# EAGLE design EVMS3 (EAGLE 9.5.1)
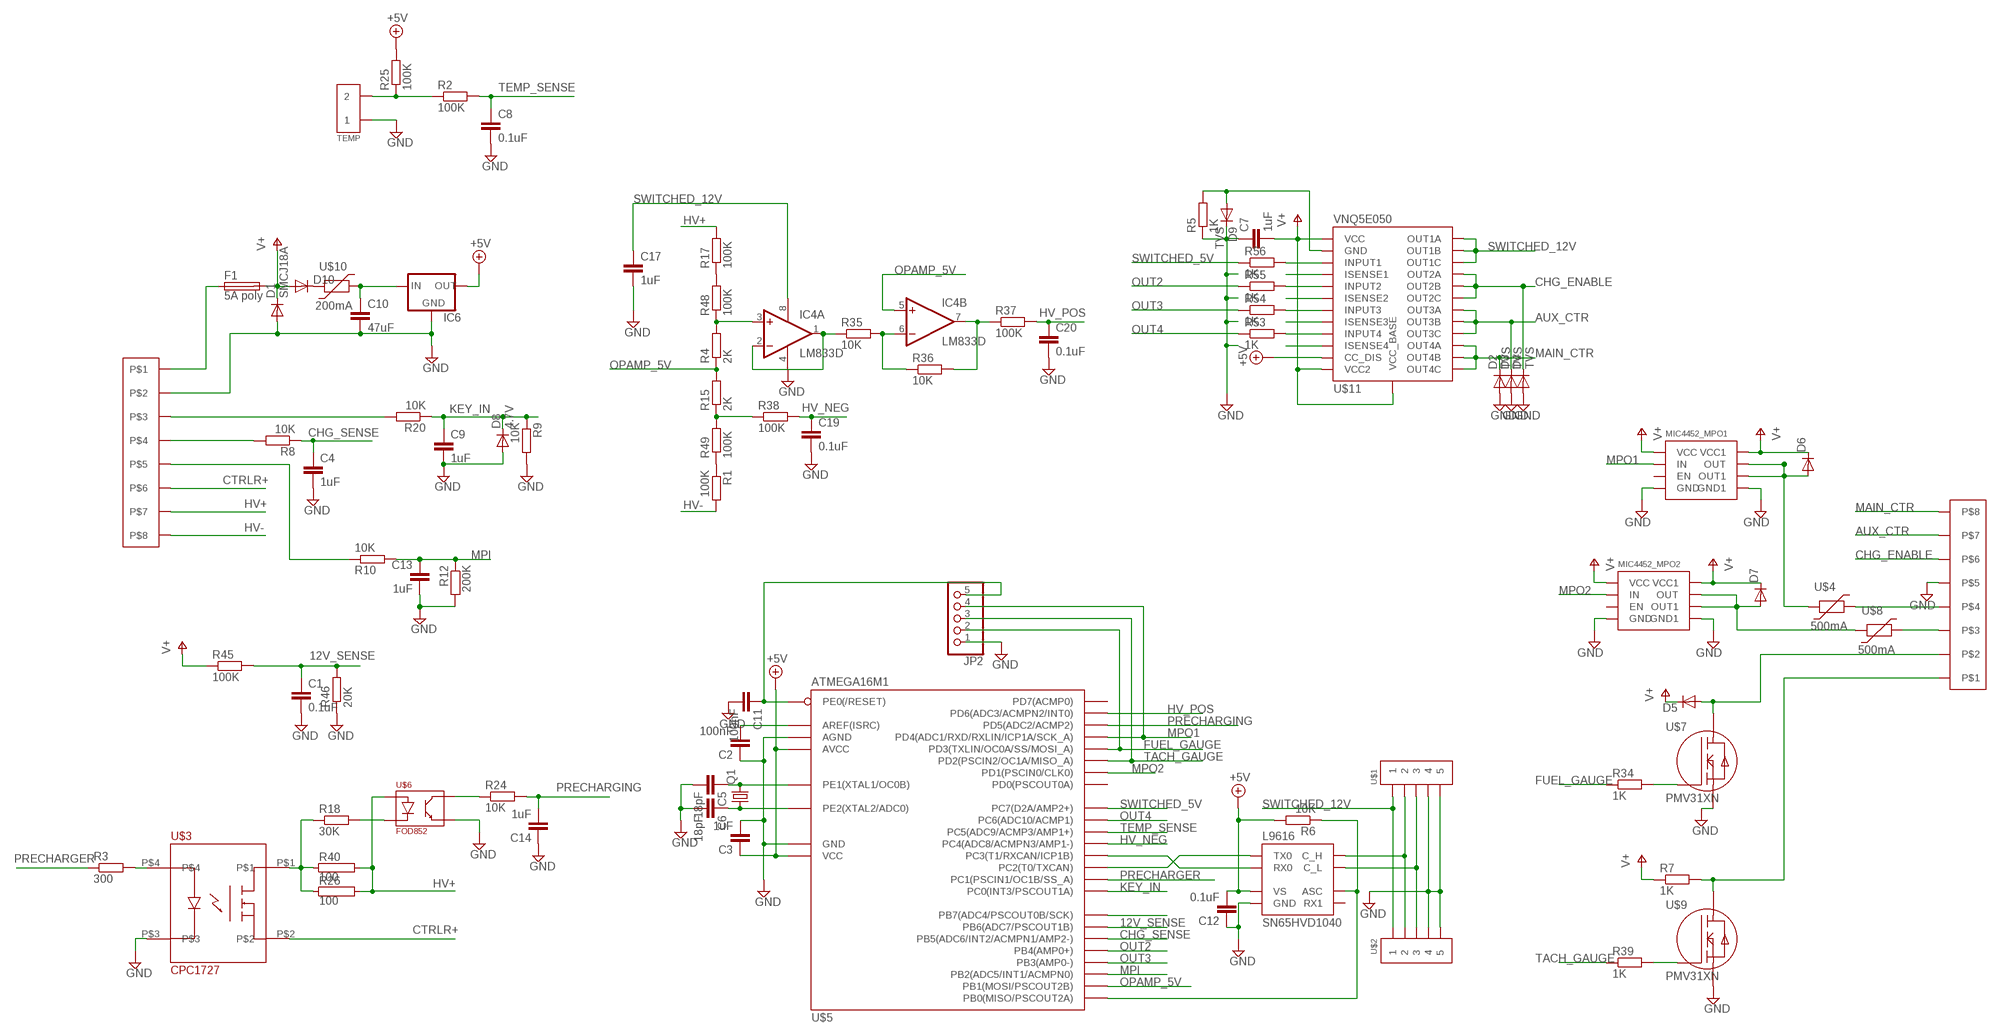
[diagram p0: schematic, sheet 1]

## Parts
C1  0.1uF  C-EUC1206  [C1206]
C2  100nF  C-EUC1206  [C1206]
C3  1uF  C-EUC1206  [C1206]
C4  1uF  C-EUC1206  [C1206]
C5  18pF  C-EUC0805  [C0805]
C6  18pF  C-EUC0805  [C0805]
C7  1uF  C-EUC1206  [C1206]
C8  0.1uF  C-EUC1206  [C1206]
C9  1uF  C-EUC1206  [C1206]
C10  47uF  C-EUC1206  [C1206]
C11  100nF  C-EUC1206  [C1206]
C12  0.1uF  C-EUC1206  [C1206]
C13  1uF  C-EUC1206  [C1206]
C14  1uF  C-EUC1206  [C1206]
C17  1uF  C-EUC1206  [C1206]
C19  0.1uF  C-EUC1206  [C1206]
C20  0.1uF  C-EUC1206  [C1206]
D1  SMCJ18A  DIODE-SMC  [SMC]
D2  TVS  DIODE-SOD123  [SOD123]
D3  TVS  DIODE-SOD123  [SOD123]
D4  TVS  DIODE-SOD123  [SOD123]
D5  DIODE-SOD123  [SOD123]
D6  DIODE-SOD123  [SOD123]
D7  DIODE-SOD123  [SOD123]
D8  4.7V  DIODE-SOD123  [SOD123]
D9  TVS  DIODE-SOD123  [SOD123]
D10  DIODE-SOD123  [SOD123]
F1  5A poly  TE5  [TE5]
IC4  LM833D  [SO08]
IC6  78LXXSOT89  [SOT89R]
JP2  PINHD-1X5  [1X05]
MIC4452_MPO1  IXDD414CI  [SOIC8]
MIC4452_MPO2  IXDD414CI  [SOIC8]
Q1  CRYSTALCTS406  [CTS406]
R1  100K  R-EU_R1206  [R1206]
R2  100K  R-EU_R1206  [R1206]
R3  300  R-EU_R1206  [R1206]
R4  2K  R-EU_R1206  [R1206]
R5  1K  R-EU_R1206  [R1206]
R6  10K  R-EU_R1206  [R1206]
R7  1K  R-EU_R1206  [R1206]
R8  10K  R-EU_R1206  [R1206]
R9  10K  R-EU_R1206  [R1206]
R10  10K  R-EU_R1206  [R1206]
R12  200K  R-EU_R1206  [R1206]
R15  2K  R-EU_R1206  [R1206]
R17  100K  R-EU_R1206  [R1206]
R18  30K  R-EU_R2512  [R2512]
R20  10K  R-EU_R1206  [R1206]
R24  10K  R-EU_R1206  [R1206]
R25  100K  R-EU_R1206  [R1206]
R26  100  RKH206-8  [KH206-8]
R34  1K  R-EU_R1206  [R1206]
R35  10K  R-EU_R1206  [R1206]
R36  10K  R-EU_R1206  [R1206]
R37  100K  R-EU_R1206  [R1206]
R38  100K  R-EU_R1206  [R1206]
R39  1K  R-EU_R1206  [R1206]
R40  100  RKH206-8  [KH206-8]
R45  100K  R-EU_R1206  [R1206]
R46  20K  R-EU_R1206  [R1206]
R48  100K  R-EU_R1206  [R1206]
R49  100K  R-EU_R1206  [R1206]
R53  1K  R-EU_R1206  [R1206]
R54  1K  R-EU_R1206  [R1206]
R55  1K  R-EU_R1206  [R1206]
R56  1K  R-EU_R1206  [R1206]
SN65HVD1040  L9616  [SOIC8]
TEMP  MOLEX-39502-1002  [MOLEX-39502-1002]
U$1  MOLEX-39502-1005  [MOLEX-39502-1005]
U$2  MOLEX-39502-1005  [MOLEX-39502-1005]
U$3  CPC1727  [CPC1727]
U$4  500mA  1206_POLYSWITCH  [1206]
U$5  ATMEGA16M1  [TQFP32]
U$6  FOD852  [SMD4]
U$7  PMV31XN  [SOT23]
U$8  500mA  1206_POLYSWITCH  [1206]
U$9  PMV31XN  [SOT23]
U$10  200mA  1206_POLYSWITCH  [1206]
U$11  VNQ5E050  [POWERSSO-24]
U$12  MOLEX-38720-6208INLINE_PINS  [MOLEX-38720-6208-B]
U$13  MOLEX-38720-6208INLINE_PINS  [MOLEX-38720-6208-B]

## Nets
12V_SENSE: C1.1 R45.2 R46.2 U$5.27(PB6(ADC7/PSCOUT1B))
+5V: C3.1 C12.2 IC6.2(OUT) R6.2 R25.2 SN65HVD1040.P$3(VS) U$5.4(VCC) U$5.19(AVCC) U$11.P$11(CC_DIS)
AUX_CTR: D3.C U$11.P$16(OUT3C) U$11.P$17(OUT3B) U$11.P$18(OUT3A) U$13.7
CHG_ENABLE: D4.C U$11.P$19(OUT2C) U$11.P$20(OUT2B) U$11.P$21(OUT2A) U$13.6
CHG_SENSE: C4.1 R8.1 U$5.26(PB5(ADC6/INT2/ACMPN1/AMP2-))
CTRLR+: U$3.P$2 U$12.6
FSA: R6.1 SN65HVD1040.P$8(ASC) U$5.8(PB0(MISO/PSCOUT2A))
FUEL_GAUGE: JP2.2 R34.1 U$5.2(PD3(TXLIN/OC0A/SS/MOSI_A))
GND: C1.2 C2.1 C3.2 C4.2 C5.2 C6.2 C7.1 C8.2 C9.2 C10.2 C11.2 C12.1 C13.2 C14.1 C17.2 C19.2 C20.2 D1.A D2.A D3.A D4.A D8.A D9.C IC4.4(P:V-) IC6.4(GND) JP2.1 MIC4452_MPO1.P$4(GND) MIC4452_MPO1.P$5(GND1) MIC4452_MPO2.P$4(GND) MIC4452_MPO2.P$5(GND1) R5.1 R9.2 R12.2 R46.1 SN65HVD1040.P$2(GND) TEMP.1 U$1.4 U$1.5 U$2.4 U$2.5 U$3.P$3 U$5.5(GND) U$5.20(AGND) U$6.P$3(EM) U$7.P$2(S) U$9.P$2(S) U$12.2 U$13.5
HV+: R17.2 R26.2 R40.2 U$6.P$1(AN) U$12.7
HV-: R1.2 U$12.8
HV_NEG: C19.1 R38.2 U$5.17(PC4(ADC8/ACMPN3/AMP1-))
HV_POS: C20.1 R37.2 U$5.14(PD6(ADC3/ACMPN2/INT0))
KEY_IN: C9.1 D8.C R9.1 R20.1 U$5.30(PC0(INT3/PSCOUT1A))
MAIN_CTR: D2.C U$11.P$13(OUT4C) U$11.P$14(OUT4B) U$11.P$15(OUT4A) U$13.8
MPI: C13.1 R10.2 R12.1 U$5.16(PB2(ADC5/INT1/ACMPN0))
MPO1: JP2.4 MIC4452_MPO1.P$2(IN) U$5.12(PD4(ADC1/RXD/RXLIN/ICP1A/SCK_A))
MPO2: MIC4452_MPO2.P$2(IN) U$5.32(PD1(PSCIN0/CLK0))
N$1: IC4.3(A:+IN) R4.2 R48.1
N$2: D9.A R5.2 U$11.P$2(GND)
N$3: C10.1 IC6.1(IN) U$10.P$2
N$4: U$4.P$2 U$13.4
N$5: R2.1 R25.1 TEMP.2
N$6: U$5.28(PB7(ADC4/PSCOUT0B/SCK))
N$7: SN65HVD1040.P$6(C_L) U$1.3 U$2.3
N$8: U$11.P$4(ISENSE1)
N$9: R18.2 U$6.P$2(CAT)
N$10: SN65HVD1040.P$7(C_H) U$1.2 U$2.2
N$11: F1.1 U$12.1
N$12: SN65HVD1040.P$1(TX0) U$5.6(PC2(T0/TXCAN))
N$13: R10.1 U$12.5
N$14: R15.1 R38.1 R49.2
N$15: D10.C U$10.P$1
N$16: R24.1 U$6.P$4(COL)
N$17: SN65HVD1040.P$4(RX0) U$5.7(PC3(T1/RXCAN/ICP1B))
N$18: U$11.P$6(ISENSE2)
N$19: U$8.P$2 U$13.3
N$21: C6.1 Q1.1 U$5.11(PE2(XTAL2/ADC0))
N$22: D6.A MIC4452_MPO1.P$6(OUT) MIC4452_MPO1.P$7(OUT1) U$4.P$1
N$25: U$11.P$8(ISENSE3)
N$26: R18.1 R26.1 R40.1 U$3.P$1
N$27: R1.1 R49.1
N$28: U$11.P$10(ISENSE4)
N$30: R3.2 U$3.P$4
N$31: R17.1 R48.2
N$32: R20.2 U$12.3
N$34: C5.1 Q1.3 U$5.10(PE1(XTAL1/OC0B))
N$35: R53.2 U$11.P$9(INPUT4)
N$37: R8.2 U$12.4
N$39: R54.2 U$11.P$7(INPUT3)
N$41: R55.2 U$11.P$5(INPUT2)
N$42: C2.2 U$5.21(AREF(ISRC))
N$43: R56.2 U$11.P$3(INPUT1)
N$44: C11.1 JP2.5 U$5.31(PE0(/RESET))
N$51: D7.A MIC4452_MPO2.P$6(OUT) MIC4452_MPO2.P$7(OUT1) U$8.P$1
N$54: D5.A U$7.P$3(D) U$13.2
N$55: R34.2 U$7.P$1(G)
N$56: R7.2 U$9.P$3(D) U$13.1
N$57: R39.2 U$9.P$1(G)
N$64: IC4.1(A:OUT) IC4.2(A:-IN) R35.1
N$65: IC4.6(B:-IN) R35.2 R36.1
N$66: IC4.7(B:OUT) R36.2 R37.1
OPAMP_5V: IC4.5(B:+IN) R4.1 R15.2 U$5.9(PB1(MOSI/PSCOUT2B))
OUT2: R55.1 U$5.24(PB4(AMP0+))
OUT3: R54.1 U$5.23(PB3(AMP0-))
OUT4: R53.1 U$5.22(PC6(ADC10/ACMP1))
PRECHARGER: R3.1 U$5.3(PC1(PSCIN1/OC1B/SS_A))
PRECHARGING: C14.2 R24.2 U$5.13(PD5(ADC2/ACMP2))
SWITCHED_5V: R56.1 U$5.25(PC7(D2A/AMP2+))
SWITCHED_12V: C17.1 IC4.8(P:V+) U$1.1 U$2.1 U$11.P$22(OUT1C) U$11.P$23(OUT1B) U$11.P$24(OUT1A)
TACH_GAUGE: JP2.3 R39.1 U$5.1(PD2(PSCIN2/OC1A/MISO_A))
TEMP_SENSE: C8.1 R2.2 U$5.18(PC5(ADC9/ACMP3/AMP1+))
V+: C7.2 D1.C D5.C D6.C D7.C D10.A F1.2 MIC4452_MPO1.P$1(VCC) MIC4452_MPO1.P$8(VCC1) MIC4452_MPO2.P$1(VCC) MIC4452_MPO2.P$8(VCC1) R7.1 R45.1 U$11.P$1(VCC) U$11.P$12(VCC2) U$11.PAD(VCC_BASE)
Unconnected: MIC4452_MPO1.P$3(EN) MIC4452_MPO2.P$3(EN) SN65HVD1040.P$5(RX1) U$5.15(PD7(ACMP0)) U$5.29(PD0(PSCOUT0A))

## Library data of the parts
C1-C14 C17 C19 C20 = resistor:C-EU: CAPACITOR, European symbol
D1-D10 = diode:DIODE-: DIODE
F1 = fuse:TE5: FUSE
IC4 = linear:LM833: OP AMP
IC6 = v-reg:78LXX: VOLTAGE REGULATOR
JP2 = pinhead:PINHD-1X5: PIN HEADER
MIC4452_MPO1 MIC4452_MPO2 = Ians parts:IXDD414CI: IXYS 14A MOSFET driver
Q1 = crystal:CRYSTAL: CRYSTAL
R1-R6 R8-R10 R12 R15 R17 R18 R20 R24 R25 R35-R38 R45 R46 R48 R49 R53-R56 = resistor:R-EU_: RESISTOR, European symbol
R7 R34 R39 = rcl:R-EU_: RESISTOR, European symbol
R26 R40 = resistor-power:R: Power Resitor
SN65HVD1040 = Ians parts:L9616
TEMP = Ians parts:MOLEX-39502-1002
U$1 U$2 = Ians parts:MOLEX-39502-1005
U$3 = Ians parts:CPC1727
U$4 U$8 U$10 = Ians parts:1206_POLYSWITCH
U$5 = Ians parts:ATMEGA16M1
U$6 = Ians parts:FOD852
U$7 U$9 = Ians parts:PMV31XN
U$11 = Ians parts:VNQ5E050
U$12 U$13 = Ians parts:MOLEX-38720-6208

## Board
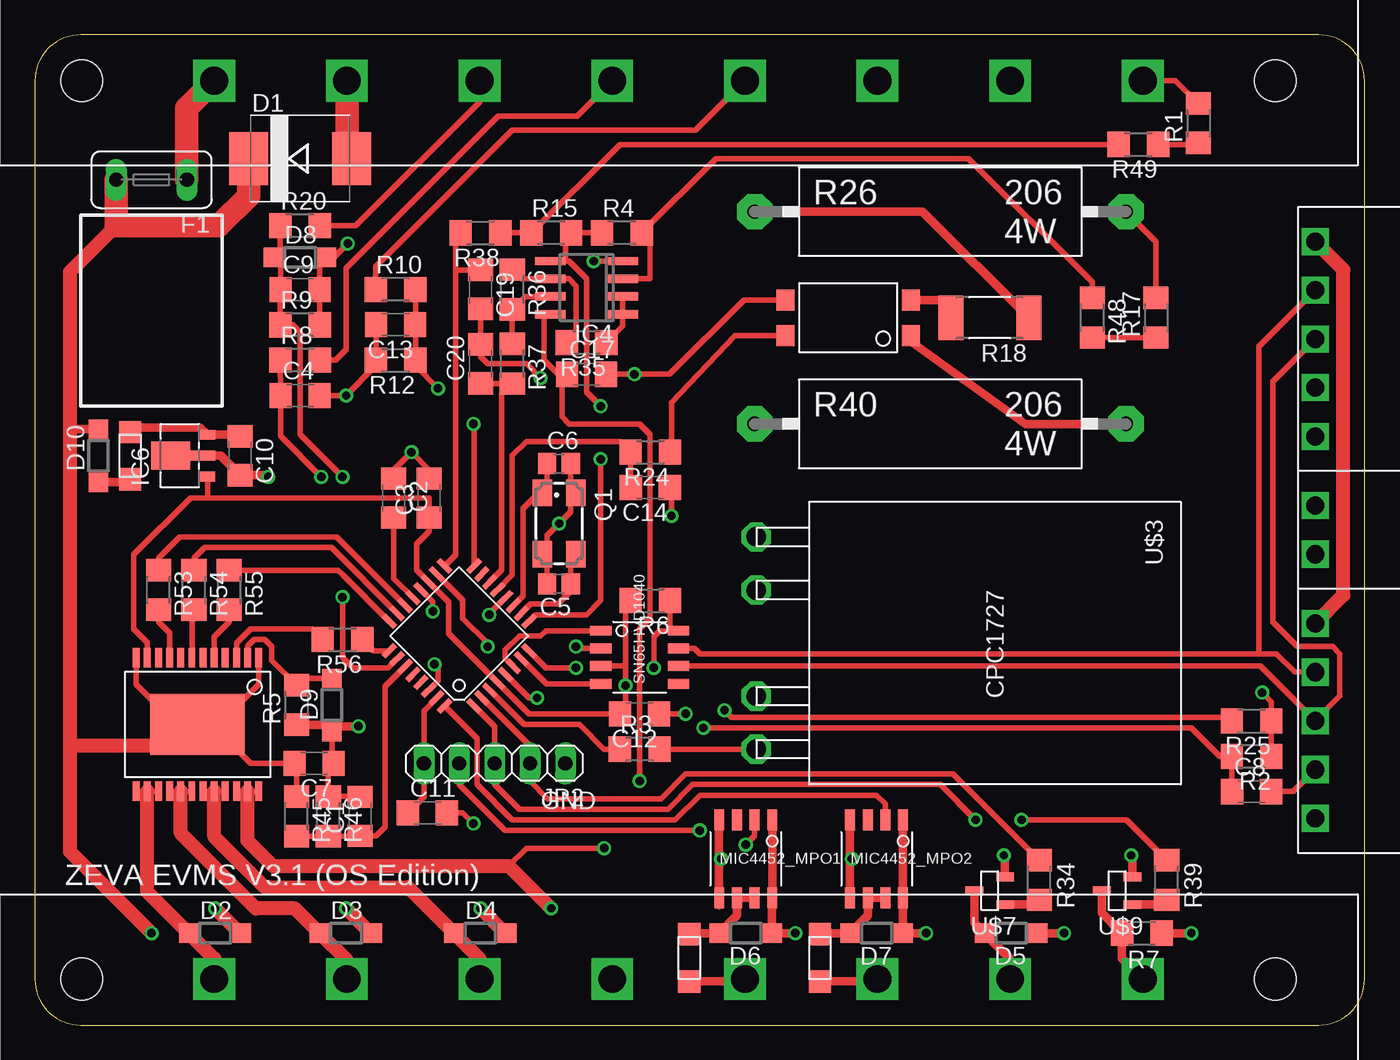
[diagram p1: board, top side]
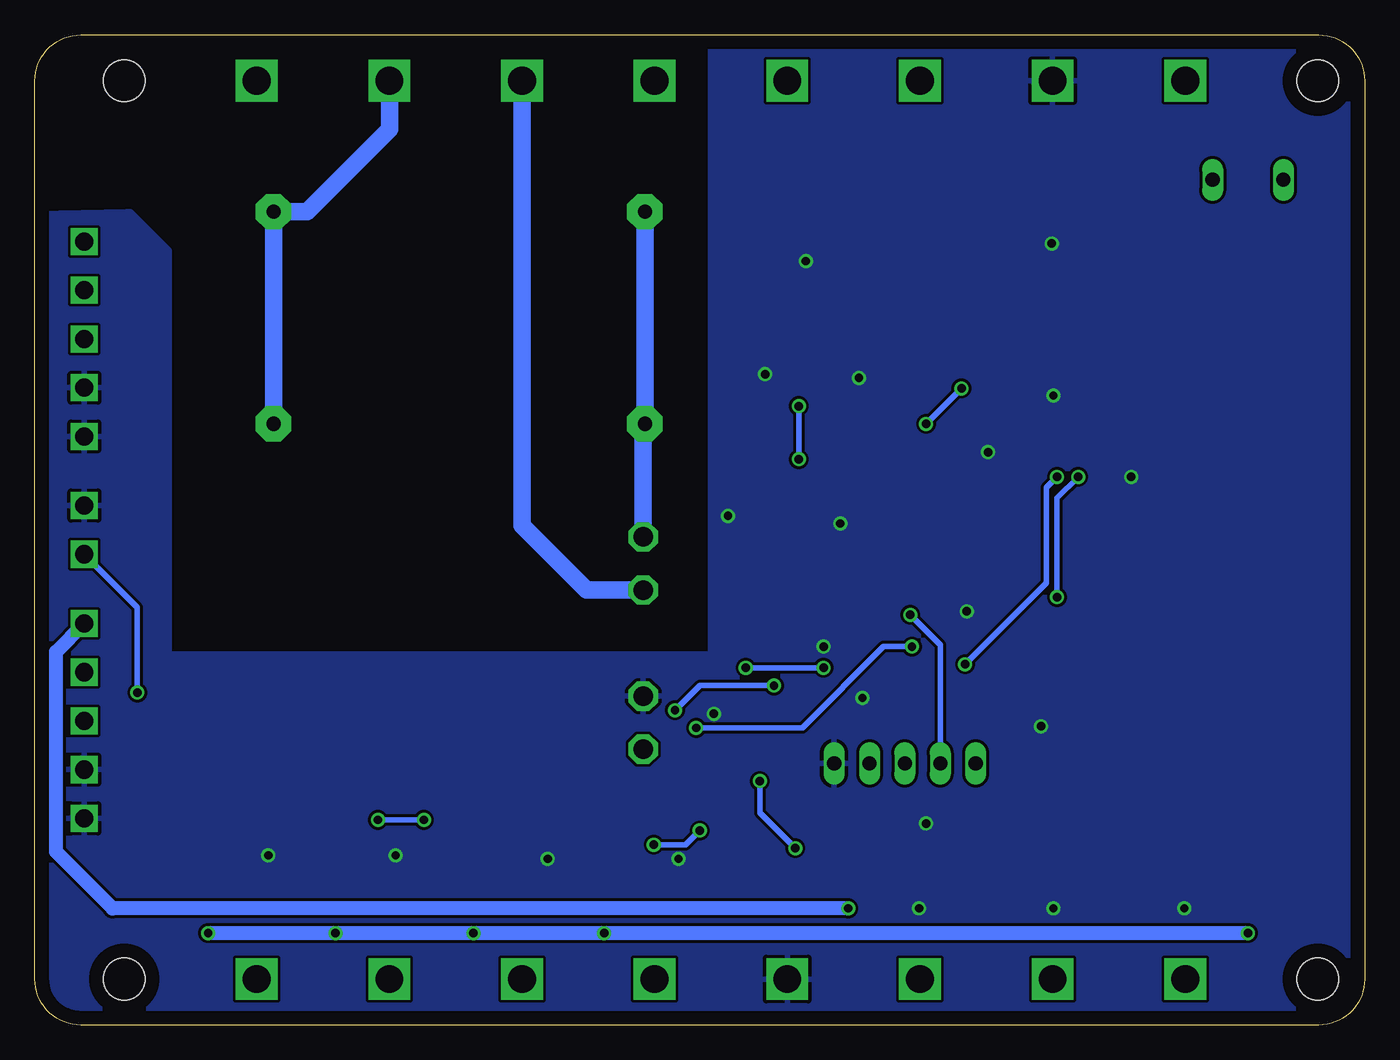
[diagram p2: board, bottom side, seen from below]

Size 95.5 x 71.12 mm. Coordinates in mm from the lower left corner, seen from the top.
Outline: 3.3,71.12 arc90 0,67.82 0,3.3 arc90 3.3,0 92.2,0 arc90 95.5,3.3 95.5,67.82 arc90 92.2,71.12 3.3,71.12
Copper layers (1*16): Top 0.035mm / dielectric 1.5mm / Bottom 0.035mm
Design rules "default *": minimum track width 10mil, minimum drill 10mil, track to track 8mil, track to pad 8mil, pad to pad 8mil, via to via 8mil, smd to smd 8mil, copper to edge 40mil, drill to drill 8mil, minimum pad ring 10mil, minimum via ring 8mil, stop-mask expansion 4mil, vias tented up to drill 0mil, thermal gap 10mil

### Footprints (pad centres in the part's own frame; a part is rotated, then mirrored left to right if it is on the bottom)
C1206 = smd 1.6 x 1.8: 1 -1.4,0; 2 1.4,0
C0805 = smd 1.3 x 1.5: 1 -0.85,0; 2 0.85,0
SMC = smd 2.8 x 3.8: A 3.7,0; C -3.7,0
SOD123 = smd 1.4 x 1.4: A 1.9,0; C -1.9,0
TE5 = drill 1.016 long: 1 -2.54,0; 2 2.54,0
SO08 = smd 0.6 x 2.2: 1 -1.905,-2.6; 2 -0.635,-2.6; 3 0.635,-2.6; 4 1.905,-2.6; 5 1.905,2.6; 6 0.635,2.6; 7 -0.635,2.6; 8 -1.905,2.6
SOT89R = smd 0.7 x 1.1: 1 1.5,-1.75; 2 -1.5,-1.75 | smd 0.7 x 1.8: 3 0,-1.4 | smd 2 x 2.8: 4 0,0.9
1X05 = drill 1.016 long: 1 -5.08,0; 2 -2.54,0; 3 0,0; 4 2.54,0; 5 5.08,0
SOIC8 = smd 1.524 x 0.711: P$1 -2.794,1.905; P$2 -2.794,0.635; P$3 -2.794,-0.635; P$4 -2.794,-1.905; P$5 2.794,-1.905; P$6 2.794,-0.635; P$7 2.794,0.635; P$8 2.794,1.905
CTS406 = smd 1.9 x 1.4: 1 -2.2,-1.2; 2 2.2,-1.2; 3 2.2,1.2; 4 -2.2,1.2
R1206 = smd 1.6 x 1.803: 1 -1.422,0; 2 1.422,0
R2512 = smd 1.8 x 3.2: 1 -2.8,0; 2 2.8,0
KH206-8 = drill 1.016 pad 2.54 octagon: 1 -13.335,0; 2 13.335,0
MOLEX-39502-1002 = drill 1.3 square: 1 -1.75,0; 2 1.75,0
MOLEX-39502-1005 = drill 1.3 square: 1 -7,0; 2 -3.5,0; 3 0,0; 4 3.5,0; 5 7,0
CPC1727 = drill 1.4 octagon: P$1 -7.62,-16.51; P$2 -3.81,-16.51; P$3 3.81,-16.51; P$4 7.62,-16.51
1206 = smd 1.6 x 1.6: P$1 -1.7,0; P$2 1.7,0
TQFP32 = smd 1.2 x 0.4: 1 -4.3,2.8; 2 -4.3,2; 3 -4.3,1.2; 4 -4.3,0.4; 5 -4.3,-0.4; 6 -4.3,-1.2; 7 -4.3,-2; 8 -4.3,-2.8; 17 4.3,-2.8; 18 4.3,-2; 19 4.3,-1.2; 20 4.3,-0.4; 21 4.3,0.4; 22 4.3,1.2; 23 4.3,2; 24 4.3,2.8 | smd 0.4 x 1.2: 9 -2.8,-4.3; 10 -2,-4.3; 11 -1.2,-4.3; 12 -0.4,-4.3; 13 0.4,-4.3; 14 1.2,-4.3; 15 2,-4.3; 16 2.8,-4.3; 25 2.8,4.3; 26 2,4.3; 27 1.2,4.3; 28 0.4,4.3; 29 -0.4,4.3; 30 -1.2,4.3; 31 -2,4.3; 32 -2.8,4.3
SMD4 = smd 1.3 x 1.5: P$1 -4.5,1.27; P$2 -4.5,-1.27; P$3 4.5,-1.27; P$4 4.5,1.27
SOT23 = smd 1.27 x 0.635: P$1 -1.1,1; P$2 -1.1,-1; P$3 1.1,0
POWERSSO-24 = smd 1.4 x 0.5: P$1 -4.8,4.4; P$2 -4.8,3.6; P$3 -4.8,2.8; P$4 -4.8,2; P$5 -4.8,1.2; P$6 -4.8,0.4; P$7 -4.8,-0.4; P$8 -4.8,-1.2; P$9 -4.8,-2; P$10 -4.8,-2.8; P$11 -4.8,-3.6; P$12 -4.8,-4.4; P$13 4.8,-4.4; P$14 4.8,-3.6; P$15 4.8,-2.8; P$16 4.8,-2; P$17 4.8,-1.2; P$18 4.8,-0.4; P$19 4.8,0.4; P$20 4.8,1.2; P$21 4.8,2; P$22 4.8,2.8; P$23 4.8,3.6; P$24 4.8,4.4 | smd 4.4 x 6.8: PAD 0,0
MOLEX-38720-6208-B = drill 2 square: 1 -33.337,0; 2 -23.812,0; 3 -14.287,0; 4 -4.763,0; 5 4.763,0; 6 14.287,0; 7 23.812,0; 8 33.337,0 | hole 3: -42.862,0; 42.862,0

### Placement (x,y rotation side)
C1  23.37,14.99 90 top
C2  25.78,37.85 270 top
C3  28.32,37.85 90 top
C4  19.05,45.21 0 top
C5  37.64,31.69 180 top
C6  37.64,40.32 0 top
C7  20.07,18.8 180 top
C8  87.38,16.76 0 top
C9  19.05,52.83 0 top
C10  14.73,40.89 270 top
C11  28.19,15.24 0 top
C12  43.43,22.35 180 top
C13  25.91,50.29 180 top
C14  44.2,38.61 180 top
C17  39.62,46.74 0 top
C19  32,52.83 270 top
C20  32,47.5 90 top
D1  19.05,62.23 0 top
D2  12.95,6.6 0 top
D3  22.35,6.6 0 top
D4  32,6.6 0 top
D5  70.1,6.6 180 top
D6  51.05,6.6 180 top
D7  60.45,6.6 180 top
D8  19.05,55.12 0 top
D9  21.34,22.99 90 top
D10  4.57,40.89 90 top
F1  8.38,60.71 180 top
IC4  39.62,52.96 90 top
IC6  10.67,40.89 90 top
JP2  33.02,18.8 180 top
MIC4452_MPO1  51.05,11.94 270 top
MIC4452_MPO2  60.45,11.94 270 top
Q1  37.66,36.02 270 top
R1  83.57,64.77 90 top
R2  87.38,19.3 180 top
R3  43.43,19.81 0 top
R4  42.16,56.9 0 top
R5  18.8,22.99 90 top
R6  44.2,30.48 180 top
R7  79.5,6.6 180 top
R8  19.05,47.75 0 top
R9  19.05,50.29 0 top
R10  25.91,52.83 0 top
R12  25.91,47.75 180 top
R15  37.08,56.9 0 top
R17  80.52,50.8 90 top
R18  68.58,50.8 180 top
R20  19.05,57.4 0 top
R24  44.2,41.15 180 top
R25  87.38,21.84 180 top
R26  65.02,58.42 0 top
R34  72.14,10.41 270 top
R35  39.62,49.02 180 top
R36  34.29,52.83 270 top
R37  34.29,47.5 270 top
R38  32,56.9 180 top
R39  81.28,10.41 270 top
R40  65.02,43.18 0 top
R45  18.8,14.99 270 top
R46  21.08,14.99 270 top
R48  75.95,50.8 270 top
R49  79.25,63.25 180 top
R53  8.89,31.24 270 top
R54  11.43,31.24 270 top
R55  13.97,31.24 270 top
R56  22.1,27.69 180 top
SN65HVD1040  43.43,26.42 0 top
TEMP  91.95,35.56 270 top
U$1  91.95,49.28 270 top
U$2  91.95,21.84 270 top
U$3  68.33,27.43 270 top
U$4  46.99,4.83 270 top
U$5  30.48,27.94 135 top
U$6  58.42,50.8 180 top
U$7  68.58,9.65 180 top
U$8  56.39,4.83 270 top
U$9  77.72,9.65 180 top
U$10  6.86,40.89 90 top
U$11  11.68,21.59 270 top
U$12  46.23,67.82 0 top
U$13  46.23,3.3 180 top

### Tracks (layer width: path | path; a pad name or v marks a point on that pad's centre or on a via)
12V_SENSE
  Top 0.406: U$5.27 25.15,24.3 25.15,14.22 24.51,13.59 C1.1 23.37,13.56 R46.2 R45.2
+5V  (via drill 0.6)
  Top 0.406: R6.2 42.42,29.82 42.42,25.78 | 42.42,25.78 v42.42,24.38 42.42,23.11 42.03,22.98 C12.2 35.5,22.35 U$5.4 29.72,28.14 29.72,30.4 U$5.19 27.43,32.69 27.43,34.54 28.32,35.43 C3.1 28.32,37.85 12.42,37.85 | 42.42,25.78 SN65HVD1040.P$3 | U$11.P$11 8.08,27.48 7.11,28.45 7.11,33.78 11.18,37.85 12.42,37.85 | 12.42,37.85 IC6.2 | R25.2 85.7,22.1 50.04,22.1 v49.53,22.61
  Bottom 0.406: v42.42,24.38 47.75,24.38 v49.53,22.61
AUX_CTR
  Top 0.406: U$11.P$18 U$11.P$17 U$11.P$16
  Top 1.016: U$11.P$17 10.48,13.77 15.88,8.38 18.67,8.38 D3.C 22.42,4.64 U$13.7
CHG_ENABLE
  Top 0.406: U$11.P$21 U$11.P$20 U$11.P$19
  Top 1.016: U$11.P$20 12.88,13.53 16.51,9.91 26.8,9.91 D4.C 31.94,4.77 U$13.6
CHG_SENSE  (via drill 0.6)
  Top 0.406: U$5.26 25.37,25.65 22.86,25.65 22.1,26.42 v22.1,30.73 | R8.1 17.63,47.77 C4.1 17.65,42.29 v20.57,39.37
  Bottom 0.406: v22.1,30.73 22.1,37.85 v20.57,39.37
CTRLR+
  Bottom 1.27: U$12.6 60.52,35.88 55.88,31.24 U$3.P$2
FSA  (via drill 0.6)
  Top 0.406: U$5.8 36.73,25.65 v38.86,25.65 | 45.62,28.32 SN65HVD1040.P$8 | 45.62,28.32 R6.1 | 45.62,28.32 44.86,28.32 44.45,27.91 v44.45,25.65
  Bottom 0.406: v38.86,25.65 v44.45,25.65
FUEL_GAUGE
  Top 0.406: U$5.2 35.56,20.03 JP2.2 35.56,17.53 36.83,16.26 44.96,16.26 46.74,18.03 65.94,18.03 R34.1
GND  (via drill 0.6)
  Top 0.406: v28.57,29.72 28.57,30.41 U$5.20 | D9.C 21.34,18.93 C7.1 21.08,18.8 R46.1 23.37,16.41 C1.2 | v40.13,54.86 IC4.4 | C2.1 25.78,39.88 v27.05,41.15 28.32,39.88 C3.2 | C6.2 38.49,36.85 v37.66,36.02 36.79,35.15 C5.2 | v36.32,46.48 35.31,47.5 32.51,47.5 32,48.01 C20.2 C19.2 | C17.2 v43.05,46.74 45.59,46.74 50.93,52.07 U$6.P$3 | v31.5,14.48 30.73,15.24 C11.2 | U$5.5 35.49,23.5 v36.07,23.5 | SN65HVD1040.P$2 38.86,27.05 v38.86,27.18 | C12.1 v46.74,22.35 | v45.72,36.58 45.72,38.48 C14.1 | v22.48,56.13 21.46,55.12 D8.A 20.47,54.64 20.47,52.85 C9.2 20.45,50.31 R9.2 | MIC4452_MPO1.P$5 49.15,8.48 | C8.2 90.37,16.76 U$2.4 | C13.2 24.51,47.77 R12.2 24.49,47.35 v22.35,45.21 C4.2
  Top 0.61: R5.1 20.86,21.57 D9.C | D9.C 21.47,21.09 | v23.24,21.46 21.34,21.46 D9.C | U$7.P$2 69.68,12.11 v69.6,12.19 | U$9.P$2 78.82,12.11 v78.74,12.19 | MIC4452_MPO1.P$5 49.15,11.81 v49.28,11.94 49.15,12.06 MIC4452_MPO1.P$4 | MIC4452_MPO2.P$5 58.55,11.81 v58.67,11.94 58.55,12.06 MIC4452_MPO2.P$4 | IC6.4 13.33,40.89 C10.2 16.64,39.49 v16.76,39.37
  Top 1.016: D2.A 14.73,6.6 v12.95,8.38 | D3.A 24.13,6.6 v22.35,8.38 | D4.A 33.78,6.6 v32,8.38
  Top 1.676: D1.A 22.42,64.05 U$12.2
  pour Bottom: -1.27,-1.27 100.33,-1.27 100.33,58.17 88.9,58.42 88.65,58.42 85.85,55.63 85.85,26.67 46.99,26.67 46.99,73.66 -1.27,73.66
HV+
  Top 0.406: R40.2 78.49,43.31 | R17.2 80.52,56.26 R26.2
  Top 0.61: U$6.P$1 62.92,49.09 71.12,43.18 R40.2
  Bottom 1.27: U$12.7 70.04,64.33 75.95,58.42 R26.2 R40.2
HV-
  Top 0.406: R1.2 81.89,67.82 U$12.8
HV_NEG
  Top 0.406: 30.23,54.23 30.23,56.54 R38.2 | 30.23,54.23 C19.1 | 30.23,54.23 30.23,33.77 U$5.17
HV_POS
  Top 0.406: U$5.14 33.53,32.69 33.53,45.31 R37.2 32.03,46.08 C20.1
KEY_IN  (via drill 0.6)
  Top 0.406: U$5.30 28.96,24.72 28.96,25.65 v28.7,25.91 | v22.1,39.37 19.05,42.42 19.05,49.78 18.54,50.29 R9.1 17.63,52.81 C9.1 17.65,54.62 D8.C 17.63,55.6 R20.1
  Bottom 0.406: v28.7,25.91 22.86,31.75 22.86,38.61 v22.1,39.37
MAIN_CTR
  Top 0.406: U$11.P$13 U$11.P$14 U$11.P$15
  Top 1.016: U$11.P$14 8.08,9.57 D2.C 12.89,4.77 U$13.8
MPI  (via drill 0.6)
  Top 0.406: U$5.16 31.54,43.13 v31.5,43.18 | v28.96,45.72 27.33,47.35 R12.1 27.33,50.27 C13.1 27.33,50.31 R10.2
  Bottom 0.406: v31.5,43.18 v28.96,45.72
MPO1  (via drill 0.6)
  Top 0.406: U$5.12 32.64,29.53 v32.64,29.46 | MIC4452_MPO1.P$2 51.69,13.59 v51.05,12.95 | JP2.4 30.48,17.27 33.78,13.97 v47.75,13.97
  Bottom 0.406: v32.64,29.46 30.48,27.3 JP2.4 | v51.05,12.95 48.77,12.95 v47.75,13.97
MPO2
  Top 0.406: MIC4452_MPO2.P$2 61.09,15.88 60.45,16.51 47.75,16.51 45.97,14.73 34.29,14.73 31.75,17.27 31.75,20.59 U$5.32
N$1
  Top 0.406: IC4.3 44.2,53.59 44.2,56.29 R4.2 48.92,62.23 67.06,62.23 75.95,53.34 R48.1
N$2
  Top 0.406: U$11.P$2 15.28,27.22 15.75,27.69 16.51,27.69 17.02,27.18 17.02,26.19 R5.2 19.27,24.89 D9.A
N$3
  Top 0.61: U$10.P$2 6.94,42.93 11.89,42.93 IC6.1 14.63,42.39 C10.1
N$4
  Top 0.61: U$4.P$2 50.99,3.13 U$13.4
N$5  (via drill 0.6)
  Top 0.406: v88.14,23.88 88.8,23.22 R25.1 R2.1
  Bottom 0.406: TEMP.2 88.14,30 v88.14,23.88
N$7
  Top 0.406: U$1.3 88.9,46.23 88.9,28.96 90.68,27.18 93.22,27.18 93.73,26.67 93.73,23.62 U$2.3 88.01,25.78 SN65HVD1040.P$6
N$9
  Top 0.61: U$6.P$2 65.78,52.07 R18.2
N$10
  Top 0.406: SN65HVD1040.P$7 47.37,27.05 47.75,26.67 84.84,26.67 87.88,26.67 | 87.88,26.67 89.15,26.67 90.48,25.34 U$2.2 | U$1.2 87.88,48.71 87.88,26.67
N$11
  Top 1.676: U$12.1 10.92,65.85 F1.1
N$12
  Top 0.406: U$5.6 33.78,26.34 33.78,26.92 34.8,27.94 36.32,27.94 36.7,28.32 SN65HVD1040.P$1
N$13
  Top 0.406: U$12.5 47.43,64.26 34.29,64.26 24.49,54.46 R10.1
N$14
  Top 0.406: R38.1 R15.1 42.01,63.25 R49.2
N$15
  Top 0.61: D10.C 6.6,38.99 U$10.P$1
N$16
  Top 0.406: U$6.P$4 50.29,49.53 45.72,44.7 45.72,41.25 R24.1
N$17
  Top 0.406: U$5.7 36.74,24.51 SN65HVD1040.P$4
N$19
  Top 0.61: U$8.P$2 60.52,3.13 U$13.3
N$21
  Top 0.406: C6.1 36.79,38.55 Q1.1 36.19,38.22 35.05,37.08 35.05,30.82 U$5.11
N$22
  Top 0.61: MIC4452_MPO1.P$7 MIC4452_MPO1.P$6 50.42,7.87 D6.A 46.99,6.6 U$4.P$1
N$26
  Top 0.61: R18.1 63.76,58.42 R26.1
  Bottom 1.27: U$3.P$1 51.82,43.05 R40.1 R26.1
N$27
  Top 0.406: R1.1 82.7,63.25 R49.1
N$30
  Top 0.406: R3.2 U$3.P$4
N$31
  Top 0.406: R48.2 R17.1
N$32
  Top 0.406: R20.2 23.05,57.4 31.94,66.29 U$12.3
N$34
  Top 0.406: Q1.3 38.49,33.45 C5.1 38.49,31.12 37.59,30.23 35.59,30.23 U$5.10
N$35
  Top 0.406: U$11.P$9 9.68,28.16 8.89,28.96 R53.2
N$37
  Top 0.406: R8.2 21.59,47.75 22.35,48.51 22.35,54.36 33.27,65.28 38.92,65.28 U$12.4
N$39
  Top 0.406: U$11.P$7 11.28,29.67 R54.2
N$41
  Top 0.406: U$11.P$5 12.88,27.87 13.97,28.96 R55.2
N$42
  Top 0.406: U$5.21 25.78,32.07 C2.2
N$43
  Top 0.406: U$11.P$3 14.48,27.44 15.49,28.45 19.91,28.45 R56.2
N$44
  Top 0.406: U$5.31 27.94,22.57 JP2.5 27.94,16.39 C11.1
N$51
  Top 0.61: MIC4452_MPO2.P$7 MIC4452_MPO2.P$6 59.82,7.87 D7.A 56.39,6.6 U$8.P$1
N$54
  Top 0.61: U$7.P$3 67.48,7.33 D5.A 70.04,4.77 U$13.2
N$55
  Top 0.61: U$7.P$1 71.8,8.65 R34.2
N$56
  Top 0.61: U$9.P$3 76.62,8.06 R7.2 78.08,4.79 U$13.1
N$57
  Top 0.61: U$9.P$1 80.94,8.65 R39.2
N$64
  Top 0.406: R35.1 42.22,50.2 IC4.1 IC4.2
N$65
  Top 0.406: R35.2 38.86,49.68 38.86,53.09 38.35,53.59 IC4.6 34.95,53.59 R36.1
N$66
  Top 0.406: IC4.7 35.2,52.32 R36.2 R37.1
OPAMP_5V  (via drill 0.6)
  Top 0.406: R4.1 R15.2 38.1,56.49 38.1,54.86 | 38.1,54.86 38.35,54.86 39.62,53.59 39.62,45.47 v40.64,44.45 | 38.1,54.86 IC4.5 | v40.64,40.64 40.64,30.48 39.62,29.46 35.96,29.46 U$5.9
  Bottom 0.406: v40.64,40.64 v40.64,44.45
OUT2
  Top 0.406: U$5.24 22.15,32.31 22.1,32.36 21.8,32.66 R55.1
OUT3
  Top 0.406: U$5.23 21.3,34.29 12.19,34.29 11.43,33.53 R54.1
OUT4
  Top 0.406: U$5.22 21.67,35.05 10.41,35.05 8.89,33.53 R53.1
PRECHARGER
  Top 0.406: U$5.3 35.13,21.59 39.12,21.59 40.89,19.81 R3.1
PRECHARGING
  Top 0.406: U$5.13 34.29,32.32 34.29,40.89 35.31,41.91 42.01,41.91 R24.2 42.8,41.13 C14.2
SWITCHED_5V
  Top 0.406: R56.1 24.33,26.88 U$5.25
SWITCHED_12V  (via drill 0.6)
  Top 0.406: U$11.P$22 U$11.P$23 U$11.P$24 | IC4.8 36.58,51.05 36.58,47.75 37.59,46.74 C17.1 37.85,46.36 37.85,43.69 38.35,43.18 43.43,43.18 44.2,42.42 44.2,29.21 43.43,28.45 v43.43,17.53 | 34.04,11.43 35.31,12.7 v40.89,12.7
  Top 1.016: U$11.P$23 15.28,13.23 17.09,11.43 34.04,11.43 v37.08,8.38 | U$1.1 93.98,54.24 93.98,30.88 U$2.1
  Bottom 0.406: v40.89,12.7 43.43,15.24 v43.43,17.53
  Bottom 1.016: v37.08,8.38 89.92,8.38 93.98,12.45 93.98,26.81 U$2.1
TACH_GAUGE  (via drill 0.6)
  Top 0.406: U$5.1 33.02,21.44 JP2.3 33.02,17.27 34.8,15.49 45.47,15.49 47.24,17.27 65.02,17.27 v67.56,14.73 | R39.1 78.38,14.73 v70.87,14.73
  Bottom 0.406: v67.56,14.73 v70.87,14.73
TEMP_SENSE  (via drill 0.6)
  Top 0.406: U$5.18 30.73,30.51 30.73,29.21 32.51,27.43 v32.51,27.18 | C8.1 85.98,19.28 R2.2 85.09,19.3 83.06,21.34 v48.01,21.34
  Bottom 0.406: v32.51,27.18 34.54,27.18 40.39,21.34 v48.01,21.34
V+  (via drill 0.6)
  Top 0.406: U$11.P$1 16.08,24.47 13.21,21.59 12.7,21.59 | U$11.PAD 12.7,21.59 | U$11.P$12 7.28,24.47 9.4,22.35 9.4,20.32 9.65,20.07 | 12.7,21.59 15.49,18.8 C7.2 18.8,18.8 R45.1
  Top 0.61: 12.7,20.32 U$11.PAD | v54.61,6.6 D6.C MIC4452_MPO1.P$8 MIC4452_MPO1.P$1 | v64.01,6.6 D7.C MIC4452_MPO2.P$8 MIC4452_MPO2.P$1 | v73.91,6.6 D5.C | v83.06,6.6 R7.1 | D10.A 2.54,42.79 2.54,43.94
  Top 1.016: 2.54,20.07 2.54,43.94 2.54,54.1 5.84,57.4 | 2.54,20.07 9.65,20.07 | v8.38,6.6 2.54,12.45 2.54,20.07
  Top 1.27: 9.65,20.07 12.45,20.07 12.7,20.32
  Top 1.676: F1.2 5.84,57.4 13.21,57.4 15.35,59.55 D1.C
  Bottom 1.016: v8.38,6.6 v54.61,6.6 v64.01,6.6 v73.91,6.6 v83.06,6.6

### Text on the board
tPlace: GND | ZEVA EVMS V3.1 (OS Edition)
